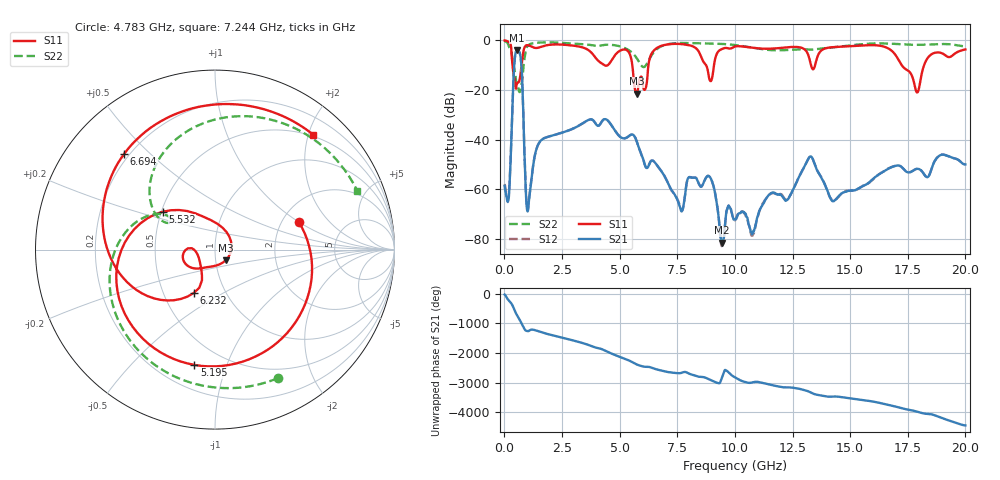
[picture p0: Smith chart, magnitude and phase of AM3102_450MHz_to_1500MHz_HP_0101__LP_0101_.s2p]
!Agilent Technologies,E8364B,MY43040894,A.07.50.67
!Agilent E8364B: A.07.50.67
!Date: Thursday, January 11, 2018 05:41:01
!Correction: S11(Full 2 Port(1,2))
!S21(Full 2 Port(1,2))
!S12(Full 2 Port(1,2))
!S22(Full 2 Port(1,2))
!S2P File: Measurements: S11, S21, S12, S22:
# Hz S  dB  R 50
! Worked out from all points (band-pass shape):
!   1601 points, 10 MHz to 20 GHz, reference 50 ohm
!   highest |S21| = -3.92 dB at 559.7 MHz (marker M1); lowest = -81.6 dB at 9.43 GHz (marker M2)
!   |S21| within 3 dB of the highest: 456.8 MHz to 705.1 MHz (248.3 MHz wide, 42.7 % of centre)
!   lowest |S11| = -21.5 dB at 5.732 GHz (marker M3), VSWR 1.18, Z = 56 - j6.61 ohm
!   |S11| at or under -10 dB: 352.1 MHz to 746.9 MHz (394.8 MHz wide, 71.8 % of centre); 5.55 GHz to 6.25 GHz (699.6 MHz wide, 11.9 % of centre); 17.24 GHz to 18.21 GHz (972.9 MHz wide, 5.49 % of centre)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
!   |S22| runs from -20.9 to -0.4 dB; largest |S21 - S12| = 0.0072
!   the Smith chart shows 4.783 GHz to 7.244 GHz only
!   S11 on the Smith chart (normalised r, x): 4.783 GHz: 2.46, +1.00; 5.195 GHz: 0.35, -0.78; 5.532 GHz: 0.51, +0.25; 6.232 GHz: 0.71, -0.37; 6.694 GHz: 0.18, +0.42; 7.244 GHz: 0.48, +2.09
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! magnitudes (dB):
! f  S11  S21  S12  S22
! 10 MHz  -0.1  -58.8  -57.9  -0.4
! 197.4 MHz  -0.7  -62.9  -61.7  -2.5
! 559.7 MHz  -17.3  -3.9  -3.9  -18.0
! 1.022 GHz  -2.0  -68.7  -68.0  -2.1
! 1.534 GHz  -2.8  -40.9  -41.0  -0.9
! 3.346 GHz  -2.7  -33.7  -33.7  -1.5
! 4.783 GHz  -6.2  -36.2  -36.2  -2.0
! 5.195 GHz  -3.7  -39.5  -39.5  -3.0
! 5.532 GHz  -8.9  -37.9  -38.0  -4.9
! 5.732 GHz  -21.5  -40.5  -40.4  -7.1
! 6.232 GHz  -11.4  -51.1  -51.0  -8.6
! 6.682 GHz  -2.7  -51.1  -51.1  -3.1
! 6.694 GHz  -2.7  -51.2  -51.3  -3.0
! 7.244 GHz  -1.5  -60.2  -60.5  -1.3
! 8.893 GHz  -15.6  -54.9  -54.9  -1.3
! 9.43 GHz  -3.6  -81.6  -83.0  -1.5
! 10.01 GHz  -2.5  -72.0  -72.6  -1.9
! 13.34 GHz  -11.1  -47.2  -47.1  -3.8
! 14.27 GHz  -2.8  -64.9  -64.5  -2.9
! 16.68 GHz  -3.4  -51.6  -51.6  -1.3
! 17.9 GHz  -21.0  -51.8  -51.7  -1.8
! 20 GHz  -3.7  -50.0  -49.9  -2.5
